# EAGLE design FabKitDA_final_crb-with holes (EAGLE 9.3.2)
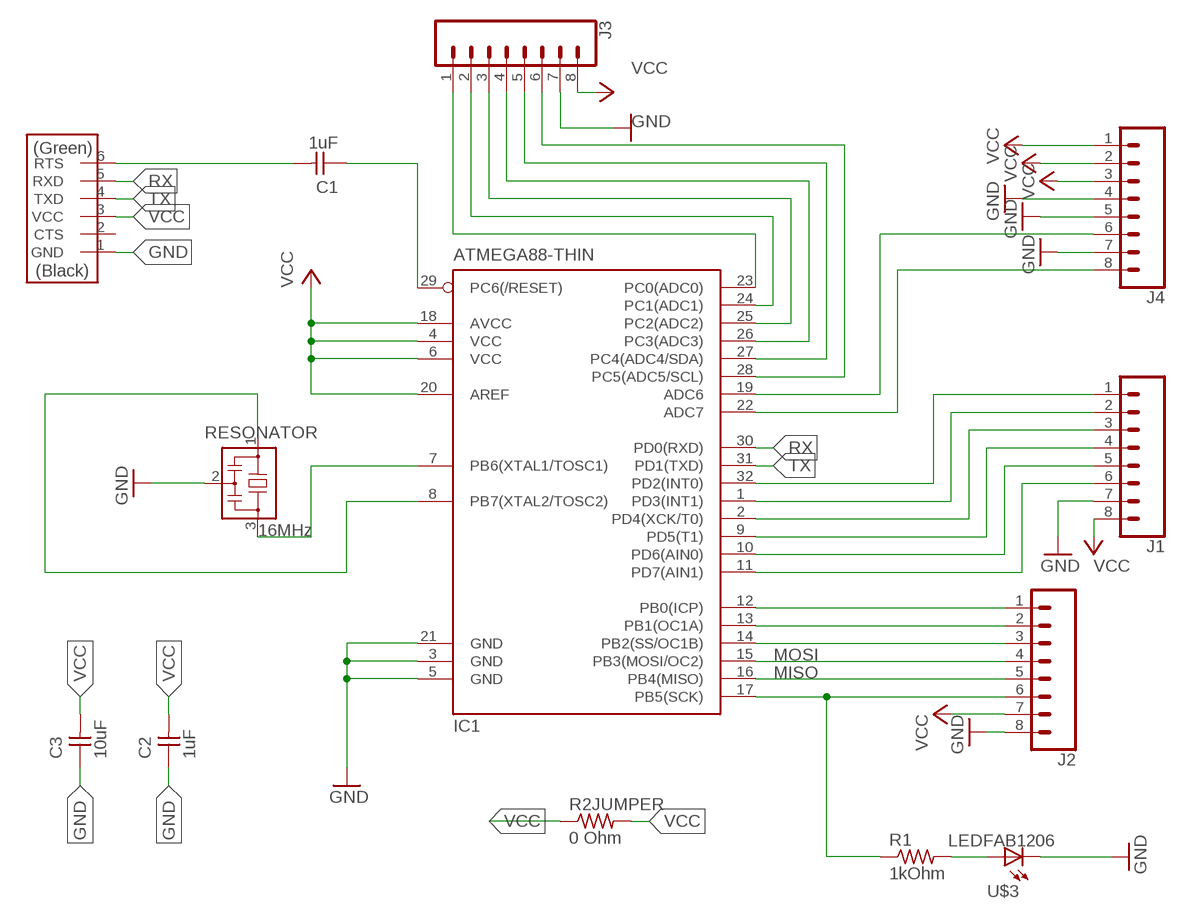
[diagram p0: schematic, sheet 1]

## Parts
C1  1uF  CAP-UNPOLARIZEDFAB  [C1206FAB]
C2  1uF  CAP-UNPOLARIZEDFAB  [C1206FAB]
C3  10uF  CAP-UNPOLARIZEDFAB  [C1206FAB]
IC1  ATMEGA88-THIN  [TQFP32-08THIN]
J1  CONN_08LONGPADS  [1X08_LONGPADS]
J2  CONN_08LONGPADS  [1X08_LONGPADS]
J3  CONN_08LONGPADS  [1X08_LONGPADS]
J4  CONN_08LONGPADS  [1X08_LONGPADS]
R1  1kOhm  RES-US1206FAB  [R1206FAB]
R2JUMPER  0 Ohm  RES-US1206FAB  [R1206FAB]
RESONATOR  16MHz  RESONATOR  [EFOBM]
U$2  FTDI-SMD-HEADER  [1X06SMD]
U$3  LEDFAB1206  [LED1206FAB]

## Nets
GND: C2.1 C3.1 IC1.3(GND) IC1.5(GND) IC1.21(GND) J1.7 J2.8 J3.7 J4.4 J4.5 J4.7 RESONATOR.2 U$2.1(GND) U$3.2(C)
MISO: IC1.16(PB4(MISO)) J2.5
MOSI: IC1.15(PB3(MOSI/OC2)) J2.4
N$1: IC1.8(PB7(XTAL2/TOSC2)) RESONATOR.1
N$2: IC1.7(PB6(XTAL1/TOSC1)) RESONATOR.3
N$3: IC1.14(PB2(SS/OC1B)) J2.3
N$4: R1.2 U$3.1(A)
N$5: IC1.17(PB5(SCK)) J2.6 R1.1
N$6: IC1.19(ADC6) J4.6
N$7: IC1.13(PB1(OC1A)) J2.2
N$8: IC1.12(PB0(ICP)) J2.1
N$9: IC1.11(PD7(AIN1)) J1.6
N$10: IC1.10(PD6(AIN0)) J1.5
N$11: IC1.9(PD5(T1)) J1.4
N$12: IC1.2(PD4(XCK/T0)) J1.3
N$13: IC1.1(PD3(INT1)) J1.2
N$14: IC1.32(PD2(INT0)) J1.1
N$15: IC1.23(PC0(ADC0)) J3.1
N$16: IC1.24(PC1(ADC1)) J3.2
N$17: IC1.25(PC2(ADC2)) J3.3
N$18: IC1.26(PC3(ADC3)) J3.4
N$19: IC1.27(PC4(ADC4/SDA)) J3.5
N$20: IC1.28(PC5(ADC5/SCL)) J3.6
N$21: IC1.22(ADC7) J4.8
RST: C1.1 C1.2 IC1.29(PC6(/RESET)) U$2.6(RTS)
RX: IC1.30(PD0(RXD)) U$2.5(RXD)
TX: IC1.31(PD1(TXD)) U$2.4(TXD)
VCC: C2.2 C3.2 IC1.4(VCC) IC1.6(VCC) IC1.18(AVCC) IC1.20(AREF) J1.8 J2.7 J3.8 J4.1 J4.2 J4.3 R2JUMPER.1 R2JUMPER.2 U$2.3(VCC)
Unconnected: U$2.2(CTS)

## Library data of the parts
C1-C3 = fab:CAP-UNPOLARIZED
IC1 = fab:ATMEGA88-THIN
J1-J4 = SparkFun-Connectors:CONN_08: Multi connection point. Often used as Generic Header-pin footprint for 0.1 inch spaced/style header connections On any of the 0.1 inch spaced packages, you can populate with these: Break Away Headers - Straight (PRT-00116) Break Away Male Headers - Right Angle (PRT-00553) Female Headers (PRT-00115)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
R1 R2JUMPER = fab:RES-US: Resistor (US Symbol)
RESONATOR = fab:RESONATOR
U$2 = fab:FTDI-SMD-HEADER
U$3 = fab:LED: LED

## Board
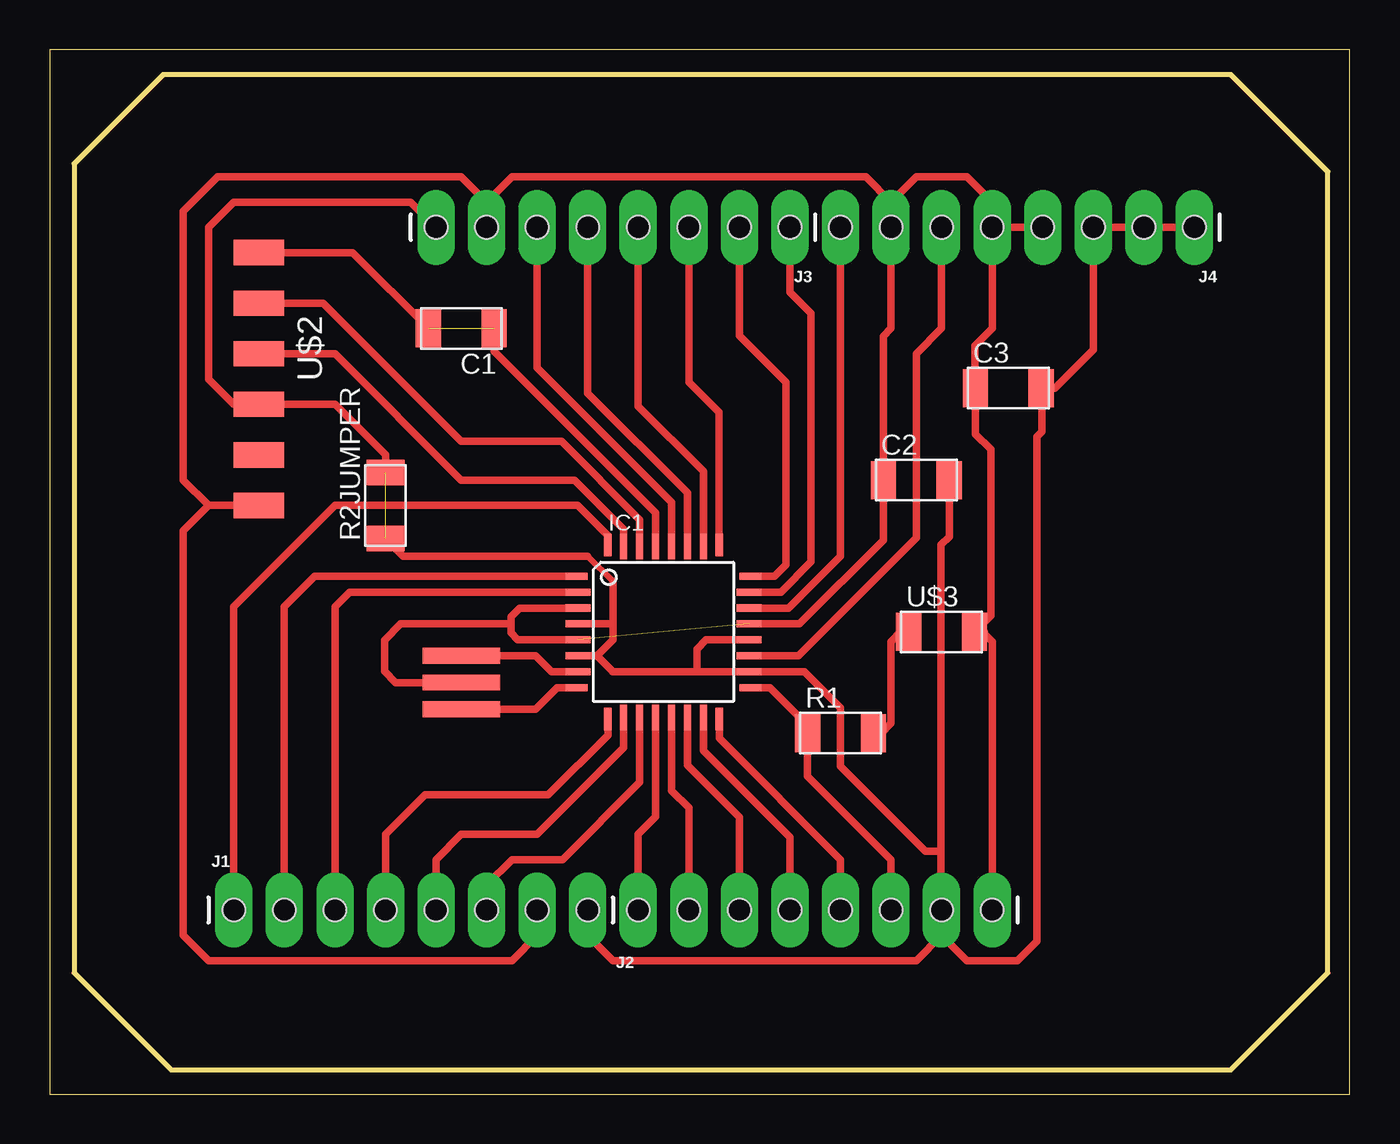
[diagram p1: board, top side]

Size 65.31 x 52.45 mm. Coordinates in mm from the lower left corner, seen from the top.
Outline: 0,0 65.31,0 65.31,52.45 0,52.45 0,0
Outline: 5.69,51.21 1.22,46.74 1.22,6.1 6.1,1.22 59.33,1.22 64.21,6.1 64.21,46.33 59.33,51.21 5.69,51.21
Copper layers (1*16): Top 0.035mm / dielectric 1.5mm / Bottom 0.035mm
Design rules "fabmodule": minimum track width 10mil, minimum drill 0.4mm, track to track 0.42mm, track to pad 0.42mm, pad to pad 0.42mm, via to via 0.42mm, smd to smd 0.42mm, copper to edge 40mil, drill to drill 0.8mm, minimum pad ring 10mil, minimum via ring 8mil, stop-mask expansion 4mil, vias tented up to drill 0mil, thermal gap 10mil
Holes 1.14 mm at 19.41,43.54 21.95,43.54 24.49,43.54 27.03,43.54 29.57,43.54 32.11,43.54 34.65,43.54 37.19,43.54 39.73,43.54 42.27,43.54 44.81,43.54 47.35,43.54 57.51,43.54 49.89,43.54 52.43,43.54 54.97,43.54 47.35,9.25 44.81,9.25 42.27,9.25 39.73,9.25 37.19,9.25 34.65,9.25 32.11,9.25 24.49,9.25 27.03,9.25 29.57,9.25 21.95,9.25 19.41,9.25 16.87,9.25 9.25,9.25 11.79,9.25 14.33,9.25

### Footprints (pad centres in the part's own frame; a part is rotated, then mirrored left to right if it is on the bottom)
C1206FAB = smd 1.27 x 1.905: 1 -1.651,0; 2 1.651,0
TQFP32-08THIN = smd 1.118 x 0.356: 1 -4.369,2.8; 8 -4.369,-2.8; 17 4.369,-2.8; 24 4.369,2.8 | smd 1.27 x 0.356: 2 -4.293,2; 3 -4.293,1.2; 4 -4.293,0.4; 5 -4.293,-0.4; 6 -4.293,-1.2; 7 -4.293,-2; 18 4.293,-2; 19 4.293,-1.2; 20 4.293,-0.4; 21 4.293,0.4; 22 4.293,1.2; 23 4.293,2 | smd 0.356 x 1.118: 9 -2.8,-4.369; 16 2.8,-4.369; 25 2.8,4.369; 32 -2.8,4.369 | smd 0.356 x 1.27: 10 -2,-4.293; 14 1.2,-4.293; 15 2,-4.293; 26 2,4.293; 27 1.2,4.293; 31 -2,4.293 | smd 0.35 x 1.27: 11 -1.2,-4.293; 12 -0.4,-4.293; 13 0.4,-4.293; 28 0.4,4.293; 29 -0.4,4.293; 30 -1.2,4.293
1X08_LONGPADS = drill 1.118 pad 1.88 long: 1 0,0; 2 2.54,0; 3 5.08,0; 4 7.62,0; 5 10.16,0; 6 12.7,0; 7 15.24,0; 8 17.78,0
R1206FAB = smd 1.27 x 1.905: 1 -1.651,0; 2 1.651,0
EFOBM = smd 0.8 x 3.9: 1 -1.35,0; 2 0,0; 3 1.35,0
1X06SMD = smd 2.54 x 1.27: 1 0,6.35; 2 0,3.81; 3 0,1.27; 4 0,-1.27; 5 0,-3.81; 6 0,-6.35
LED1206FAB = smd 1.27 x 1.905: 1 -1.651,0; 2 1.651,0

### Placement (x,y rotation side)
C1  20.68,38.46 180 top
C2  43.54,30.84 0 top
C3  48.16,35.46 0 top
IC1  30.84,23.22 0 top
J1  9.25,9.25 0 top
J2  29.57,9.25 0 top
J3  37.19,43.54 180 top
J4  57.51,43.54 180 top
R1  39.73,18.14 0 top
R2JUMPER  16.87,29.57 90 top
RESONATOR  20.68,20.68 90 top
U$2  10.52,35.92 180 top
U$3  44.81,23.22 0 top

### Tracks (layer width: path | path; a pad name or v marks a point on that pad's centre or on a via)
GND  (1 unrouted)
  Top 0.368: 7.98,29.57 U$2.1 | J1.7 24.49,7.98 23.22,6.71 7.98,6.71 6.71,7.98 6.71,28.3 7.98,29.57 | IC1.21 37.68,23.62 41.88,27.82 C2.1 41.88,38.07 42.27,38.46 J4.7 42.27,44.81 | 46.96,23.22 U$3.2 | 46.08,22.83 U$3.2 | 7.98,29.57 6.71,30.84 6.71,44.35 8.43,46.08 20.68,46.08 21.95,44.81 | 21.95,44.81 23.22,46.08 41,46.08 42.27,44.81 | J3.7 21.95,44.81 | 42.27,44.81 43.54,46.08 46.08,46.08 47.35,44.81 J4.5 | U$3.2 47.27,24.03 47.27,32.38 46.51,33.15 C3.1 46.48,35.48 46.48,37.59 47.35,38.46 J4.5 | U$3.2 46.86,23.22 47.35,22.73 J2.8 | IC1.5 23.51,22.82 23.16,23.16 23.16,23.62 | IC1.3 23.6,24.42 23.16,23.98 23.16,23.62 | RESONATOR.2 17.37,20.68 16.81,21.23 16.81,22.81 17.63,23.62 23.16,23.62 | J4.4 J4.5
MISO
  Top 0.368: IC1.16 33.64,17.88 39.73,11.79 J2.5
MOSI
  Top 0.368: IC1.15 32.84,17.25 37.19,12.9 J2.4
N$1
  Top 0.368: RESONATOR.1 24.41,19.33 25.5,20.42 IC1.8
N$2
  Top 0.368: RESONATOR.3 24.41,22.03 25.22,21.22 IC1.7
N$3
  Top 0.368: IC1.14 32.04,16.53 34.65,13.92 J2.3
N$4
  Top 0.368: 41.38,18.52 R1.2 41.78,18.14 42.27,18.62 42.27,22.73 42.75,23.22 U$3.1
N$5
  Top 0.368: IC1.17 36.18,20.42 38.07,18.52 R1.1 38.07,15.98 42.27,11.79 J2.6
N$6
  Top 0.368: J4.6 44.81,38.46 43.54,37.19 43.54,27.94 37.61,22.02 IC1.19
N$7
  Top 0.368: IC1.13 31.24,15.25 32.11,14.38 J2.2
N$8
  Top 0.368: IC1.12 30.44,13.93 29.57,13.06 J2.1
N$9
  Top 0.368: J1.6 21.95,10.52 23.22,11.79 25.76,11.79 29.64,15.67 IC1.11
N$10
  Top 0.368: IC1.10 28.84,17.41 24.49,13.06 20.68,13.06 19.41,11.79 J1.5
N$11
  Top 0.368: IC1.9 28.04,18.03 25.04,15.04 18.85,15.04 16.87,13.06 J1.4
N$12
  Top 0.368: IC1.2 15.06,25.22 14.33,24.49 J1.3
N$13
  Top 0.368: IC1.1 13.32,26.02 11.79,24.49 J1.2
N$14
  Top 0.368: J1.1 9.25,24.49 14.33,29.57 26.52,29.57 28.04,28.05 IC1.32
N$15
  Top 0.368: IC1.23 36.73,25.22 38.25,26.74 38.25,39.22 37.19,40.28 J3.1
N$16
  Top 0.368: IC1.24 36.41,26.02 36.98,26.59 36.98,35.76 34.65,38.1 J3.2
N$17
  Top 0.368: IC1.25 33.63,34.24 32.11,35.76 J3.3
N$18
  Top 0.368: IC1.26 32.84,31.27 29.57,34.54 J3.4
N$19
  Top 0.368: IC1.27 32.04,30.19 27.03,35.2 J3.5
N$20
  Top 0.368: IC1.28 31.24,29.72 24.49,36.47 J3.6
N$21
  Top 0.368: IC1.22 37.12,24.42 39.73,27.03 J4.8
RST  (1 unrouted)
  Top 0.368: U$2.6 15.21,42.27 C1.2 | 22.33,37.62 C1.1 22.33,37.31 30.44,29.2 IC1.29
RX
  Top 0.368: U$2.5 13.73,39.73 20.68,32.78 25.71,32.78 29.64,28.85 IC1.30
TX
  Top 0.368: U$2.4 14.33,37.19 20.68,30.84 26.38,30.84 28.84,28.38 IC1.31
VCC  (1 unrouted)
  Top 0.254: 26.95,22.02 IC1.6
  Top 0.33: 28.3,25.76 27.03,27.03
  Top 0.368: 44.81,7.98 J2.7 44.78,9.27 44.78,12.19 | C3.2 49.81,35.84 | J1.8 27.03,7.98 28.3,6.71 43.54,6.71 44.81,7.98 | 28.3,23.57 28.3,25.76 | R2JUMPER.2 16.87,32.11 14.33,34.65 U$2.3 9.25,34.65 7.98,35.92 7.98,43.54 9.25,44.81 18.14,44.81 J3.8 | R2JUMPER.1 17.75,27.03 27.03,27.03 | 44.81,7.98 46.08,6.71 48.62,6.71 49.58,7.67 49.58,33.02 49.83,33.27 49.83,35.43 C3.2 | C2.2 45.19,27.99 44.78,27.58 44.78,12.19 | 28.3,21.22 28.28,21.22 | 27.5,22.02 IC1.6 | 28.3,23.57 28.3,22.82 27.5,22.02 | 28.3,23.57 28.25,23.62 IC1.4 | 28.3,21.22 27.5,22.02 | C3.2 50.5,35.46 52.43,37.39 J4.3 J4.2 J4.1 | 44.78,12.19 43.99,12.19 39.73,16.46 39.73,19.41 37.92,21.22 IC1.18 32.51,21.22 | 32.51,21.22 28.3,21.22 | IC1.20 32.98,22.82 32.51,22.35 32.51,21.22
